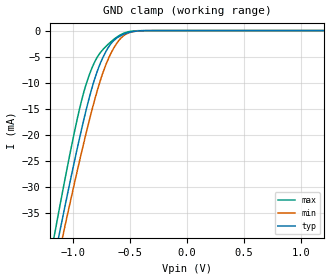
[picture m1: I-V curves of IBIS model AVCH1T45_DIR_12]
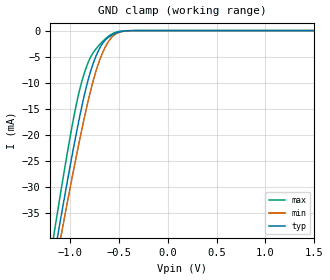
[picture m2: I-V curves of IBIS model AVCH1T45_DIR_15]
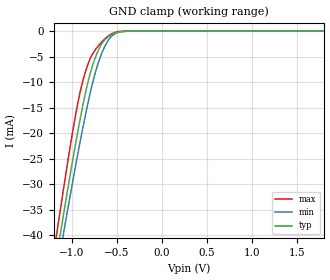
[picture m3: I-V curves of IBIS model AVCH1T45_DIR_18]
| TEXAS INSTRUMENTS INCORPORATED
| Standard Linear and Logic Group
| IBIS Model of SN74AVCH1T45
| SINGLE-BIT DUAL-SUPPLY BUS TRANSCEIVER WITH CONFIGURABLE VOLTAGE
| TRANSLATION AND 3-STATE OUTPUTS
| This file contains package information for the following:
|  SOT 6-pin (DBV) package as [Component] AVCH1T45_DBV
|  SOT 6-pin (DCK) package as [Component] AVCH1T45_DCK
|  DSBGA 6-pin (YEP_YZP) package as [Component] AVCH1T45_YEP_YZP
| This device can be powered at the following Vccs:
|  1.2 volt Vcc
|  1.5 volt Vcc
|  1.8 volt Vcc
|  2.5 volt Vcc
|  3.3 volt Vcc
| This file provides unique models under the [Model Selector] for each Vcc.
| For operation at a specific Vcc, select the appropriate model after each
| [Model Selector] keyword.
[IBIS Ver]   3.2
[Comment char]  |_char
[File Name]   sn74avch1t45.ibs
[File Rev]   1.2 | x_die
[Date]   08/31/04
[Source]   Data created from TI-SPICE simulations at TI-SLL.
[Notes]   The following is an IBIS list for the AVCH1T45.
   Please contact sllibis@ti.com with questions and
   comments concerning SLL IBIS models.
   - FILE REV HISTORY
   - 1.1 Release of IBIS File on 04/27/04
   - 1.2 YEP and YZP packages released on 08/31/04
   - Power clamp data deleted as there is no power-clamp diode.
   - Due to the fact that the Device is 4.6-V Input/Output
   tolarent, the I/O models has some Non-Monotonic Warnings.
   - Non-monotonic data in ground-clamp due to bus-hold
[Disclaimer] Property of Texas Instruments Incorporated.  Unauthorized
   reproduction and/or distribution is strictly prohibited.
   This product is protected under copyright law.
   Created  2004, (C) Copyright  2004, Texas Instruments
   Incorporated, All Rights Reserved
   UNLESS THERE IS A SIGNED, WRITTEN AGREEMENT TO THE
   CONTRARY, TEXAS INSTRUMENTS (TI) IS PROVIDING THE IBIS
   MODELS  AND WITHOUT ANY WARRANTY, EXPRESSED OR
   IMPLIED.  TI assumes no liability for:
   1) the accuracy of the IBIS models provided to your
   company;
   2) the proper functioning of these IBIS Models in your
   design or for any resulting applications; or
   3) infringement of patents, copyrights or intellectual
   property rights resulting from your use of these IBIS
   models.
   TI provides IBIS Models as a service to our customers.
   You and your company shall not distribute, sell or give
   these models to anyone else without prior written
   permission from TI.
   TI reserves the right to make changes to our products or
   to discontinue any semiconductor product or service
   without notice, and advises our customers to obtain the
   latest version of relevant information to verify, before
   placing orders, that the information being relied on is
   current.
   Please be aware that your receipt and use of the IBIS
   information provided shall serve as acceptance of these
   terms and conditions.  If you do not accept these terms,
   you should return or destroy the IBIS models and any
   other accompanying information immediately.
| Component AVCH1T45_DBV 6-pin SOT
[Component]   AVCH1T45_DBV
[Manufacturer]   Texas Instruments, Inc.
[Package]
|   typ   min   max
R_pkg   2.500e-02   1.900e-02   3.700e-02
L_pkg   1.524e-09   1.260e-09   1.751e-09
C_pkg   2.450e-13   1.980e-13   2.640e-13
[Pin]   signal_name   model_name   R_pin   L_pin   C_pin
1   VCCA   POWER   2.100e-02   1.405e-09   2.460e-13
2   GND   GND   3.700e-02   1.751e-09   2.630e-13
3   A   AVCH1T45_IOA   2.600e-02   1.493e-09   2.470e-13
4   B   AVCH1T45_IOB   1.900e-02   1.620e-09   2.640e-13
5   DIR   AVCH1T45_DIR   2.400e-02   1.260e-09   1.980e-13
6   VCCB   POWER   2.100e-02   1.617e-09   2.500e-13
| Component AVCH1T45_DCK 6-pin SOT
[Component]   AVCH1T45_DCK
[Manufacturer]   Texas Instruments, Inc.
[Package]
|   typ   min   max
R_pkg   1.400e-02   1.100e-02   2.100e-02
L_pkg   9.480e-10   7.840e-10   1.103e-09
C_pkg   1.910e-13   1.670e-13   2.050e-13
[Pin]   signal_name   model_name   R_pin   L_pin   C_pin
1   VCCA   POWER   1.300e-02   9.840e-10   1.960e-13
2   GND   GND   2.100e-02   1.103e-09   2.050e-13
3   A   AVCH1T45_IOA   1.100e-02   9.980e-10   1.970e-13
4   B   AVCH1T45_IOB   1.300e-02   9.040e-10   1.900e-13
5   DIR   AVCH1T45_DIR   1.500e-02   7.840e-10   1.670e-13
6   VCCB   POWER   1.200e-02   9.160e-10   1.950e-13
| Component AVCH1T45_YEP_YZP 6-pin DSBGA
[Component]   AVCH1T45_YEP_YZP
[Manufacturer]   Texas Instruments, Inc.
[Package]
|   typ   min   max
R_pkg   1.000e-03   1.000e-03   2.100e-02
L_pkg   2.450e-11   2.400e-11   1.103e-09
C_pkg   5.600e-14   0.000e+00   2.050e-13
[Pin]   signal_name   model_name   R_pin   L_pin   C_pin
1   VCCA   POWER   1.000e-03   2.500e-11   6.400e-14
2   GND   GND   1.000e-03   2.400e-11   6.700e-14
3   A   AVCH1T45_IOA   1.000e-03   2.500e-11   6.400e-14
4   B   AVCH1T45_IOB   1.000e-03   2.500e-11   6.400e-14
5   DIR   AVCH1T45_DIR   1.000e-03   2.400e-11   6.700e-14
6   VCCB   POWER   1.000e-03   2.500e-11   6.400e-14
| Model AVCH1T45_DIR
[Model Selector]   AVCH1T45_DIR
AVCH1T45_DIR_12   1.2 volt Vcc
AVCH1T45_DIR_15   1.5 volt Vcc
AVCH1T45_DIR_18   1.8 volt Vcc
AVCH1T45_DIR_25   2.5 volt Vcc
AVCH1T45_DIR_33   3.3 volt Vcc
| Model AVCH1T45_IOA
[Model Selector]   AVCH1T45_IOA
AVCH1T45_IOA_12   1.2 volt Vcc
AVCH1T45_IOA_15   1.5 volt Vcc
AVCH1T45_IOA_18   1.8 volt Vcc
AVCH1T45_IOA_25   2.5 volt Vcc
AVCH1T45_IOA_33   3.3 volt Vcc
| Model AVCH1T45_IOB
[Model Selector]   AVCH1T45_IOB
AVCH1T45_IOB_12   1.2 volt Vcc
AVCH1T45_IOB_15   1.5 volt Vcc
AVCH1T45_IOB_18   1.8 volt Vcc
AVCH1T45_IOB_25   2.5 volt Vcc
AVCH1T45_IOB_33   3.3 volt Vcc
| Models and submodels in the file (15): AVCH1T45_DIR_12 (Input), AVCH1T45_DIR_15 (Input), AVCH1T45_DIR_18 (Input), AVCH1T45_DIR_25 (Input), AVCH1T45_DIR_33 (Input), AVCH1T45_IOA_12 (I/O), AVCH1T45_IOA_15 (I/O), AVCH1T45_IOA_18 (I/O), AVCH1T45_IOA_25 (I/O), AVCH1T45_IOA_33 (I/O), AVCH1T45_IOB_12 (I/O), AVCH1T45_IOB_15 (I/O), AVCH1T45_IOB_18 (I/O), AVCH1T45_IOB_25 (I/O), AVCH1T45_IOB_33 (I/O)
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[Model]   AVCH1T45_DIR_12
Model_type  Input
Vinl=0.385
Vinh=0.845
| variable   typ   min   max
C_comp   2.46pF   2.11pF   2.89pF
[Temperature Range]   40   100   -40
| Ambient temperature   25   85   -40
[Voltage range]   1.2   1.1   1.3
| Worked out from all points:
|   GND clamp passes 1 mA (typ) near -0.58 V on its own axis
[GND Clamp]
| AVCH1T45_DIR_12
|   Voltage   I(typ)   I(min)   I(max)
-4.6V     -459.2mA   -437.9mA   -484.2mA
-1.165V   -43.78mA   -47mA      -39.35mA
-1.115V   -38.35mA   -41.89mA   -33.51mA
-1.09V    -35.67mA   -39.36mA   -30.63mA
-1.065V   -33.02mA   -36.85mA   -27.8mA
-945mV    -20.79mA   -25.16mA   -15.18mA
-840mV    -11.44mA   -15.71mA   -7.485mA
-710mV    -3.942mA   -6.433mA   -2.997mA
-630mV    -1.665mA   -2.889mA   -1.475mA
-555mV    -700.6uA   -964.8uA   -509.7uA
-385mV    -23.61uA   -32.06uA   -5.101uA
1.2V      106.8pA    765.6pA    17.5pA
[Model]   AVCH1T45_DIR_15
Model_type  Input
Vinl=0.49
Vinh=1.04
| variable   typ   min   max
C_comp   2.41pF   2.01pF   2.90pF
[Temperature Range]   40   100   -40
| Ambient temperature   25   85   -40
[Voltage range]   1.5   1.4   1.6
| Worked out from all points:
|   GND clamp passes 1 mA (typ) near -0.58 V on its own axis
[GND Clamp]
| AVCH1T45_DIR_15
|   Voltage   I(typ)   I(min)   I(max)
-4.6V     -459.2mA   -437.9mA   -484.2mA
-1.175V   -44.87mA   -48.03mA   -40.53mA
-1.145V   -41.6mA    -44.95mA   -37mA
-1.12V    -38.89mA   -42.4mA    -34.09mA
-1.095V   -36.21mA   -39.87mA   -31.21mA
-1.07V    -33.55mA   -37.35mA   -28.36mA
-945mV    -20.79mA   -25.16mA   -15.18mA
-840mV    -11.44mA   -15.71mA   -7.485mA
-775mV    -7.058mA   -10.58mA   -4.657mA
-700mV    -3.56mA    -5.9mA     -2.784mA
-545mV    -612.9uA   -811.6uA   -423.5uA
1.5V      118pA      793.8pA    21.88pA
[Model]   AVCH1T45_DIR_18
Model_type  Input
Vinl=0.5775
Vinh=1.2675
| variable   typ   min   max
C_comp   2.36pF   1.92pF   2.90pF
[Temperature Range]   40   100   -40
| Ambient temperature   25   85   -40
[Voltage range]   1.8   1.65   1.95
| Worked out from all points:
|   GND clamp passes 1 mA (typ) near -0.58 V on its own axis
[GND Clamp]
| AVCH1T45_DIR_18
|   Voltage   I(typ)   I(min)   I(max)
-4.6V     -459.2mA   -437.9mA   -484.2mA
-1.185V   -45.97mA   -49.06mA   -41.71mA
-1.155V   -42.69mA   -45.98mA   -38.17mA
-1.13V    -39.97mA   -43.42mA   -35.25mA
-1.105V   -37.28mA   -40.88mA   -32.35mA
-1.08V    -34.61mA   -38.36mA   -29.5mA
-950mV    -21.28mA   -25.63mA   -15.65mA
-840mV    -11.44mA   -15.71mA   -7.485mA
-765mV    -6.504mA   -9.869mA   -4.351mA
-695mV    -3.38mA    -5.644mA   -2.68mA
-540mV    -571.7uA   -743.1uA   -384.3uA
1.8V      129.6pA    822.2pA    26.26pA
